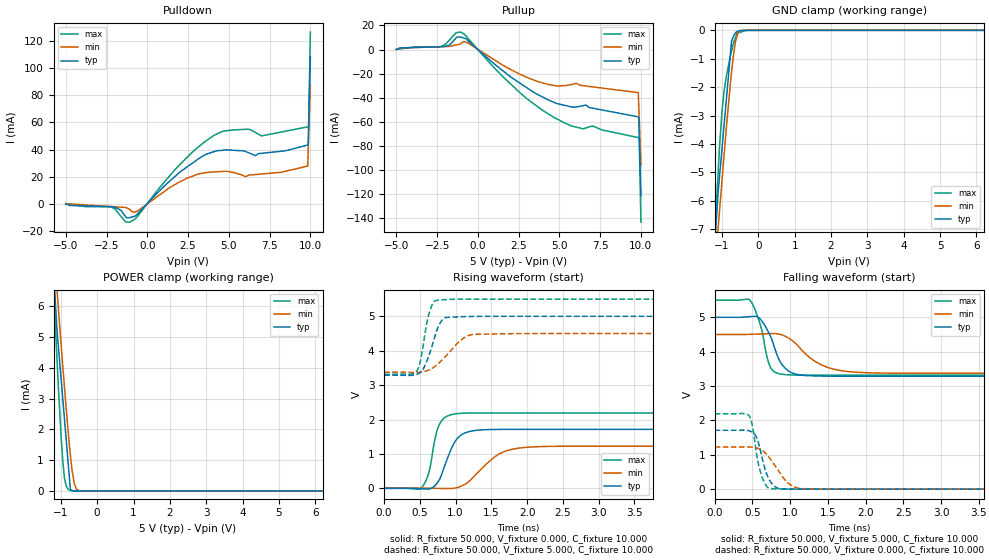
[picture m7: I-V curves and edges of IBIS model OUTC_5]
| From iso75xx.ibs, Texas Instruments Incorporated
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|   OUTC_5 MODEL
[Model]   OUTC_5
Model_type   3-state
Polarity   Non-Inverting
Vmeas = 2.5
Vref = 2.5
Cref = 15pF
Rref = 50
|   typ   min   max
| High state   (typ PVT)   (Fast PVT)  (Slow PVT)
C_comp   1.5194p   1.2464p   1.8503p
|C_comp (Low state)   1.4779p   1.2343p   1.7765p
[Voltage Range]   5   4.5   5.5
[Temperature Range]   27   125   -40
[Pullup Reference]   5   4.5   5.5
[Pulldown Reference]   -0   -0   -0
[Power Clamp Reference]   5   4.5   5.5
[GND Clamp Reference]   -0   -0   -0
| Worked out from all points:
|   slope of the pulldown table from 0 to 0.75 V, typ, clamps not added: 79.5 ohm
|   slope of the pullup table from 0 to 0.75 V, typ, clamps not added: 84.1 ohm
|   GND clamp passes 1 mA (typ) near -0.78 V on its own axis
|   POWER clamp passes 1 mA (typ) near -0.80 V on its own axis
|   falling waveform, R_fixture 50.000, V_fixture 5.000, C_fixture 10.000: 20-80 % time 200ps typ, 381ps min, 143ps max; typ from 5 V to 3.29 V
|   rising waveform, R_fixture 50.000, V_fixture 0.000, C_fixture 10.000: 20-80 % time 202ps typ, 383ps min, 130ps max; typ from 0 V to 1.71 V
|   rising waveform, R_fixture 50.000, V_fixture 5.000, C_fixture 10.000: 20-80 % time 166ps typ, 311ps min, 114ps max; typ from 3.29 V to 5 V
|   falling waveform, R_fixture 50.000, V_fixture 0.000, C_fixture 10.000: 20-80 % time 132ps typ, 241ps min, 108ps max; typ from 1.71 V to 0 V
[Pulldown]
|   Voltage   I(typ)   I(min)   I(max)
-5V       -93.83uA   -72.15uA   -88.32uA
-2.275V   -2.321mA   -2.154mA   -2.283mA
-1.07V    -10.42mA   -4.455mA   -13.77mA
-627mV    -8.011mA   -5.787mA   -9.836mA
2.106V    24.33mA    16.74mA    30.13mA
4.14V     38.62mA    23.45mA    50.79mA
6.625V    35.45mA    21.48mA    52.63mA
7.006V    37.17mA    21.87mA    50.06mA
9.838V    43.29mA    27.78mA    56.76mA
9.862V    43.37mA    36.98mA    56.82mA
9.896V    59.33mA    49.4mA     56.89mA
10V       108.8mA    87.9mA     126.9mA
[GND Clamp]
|   Voltage   I(typ)   I(min)   I(max)
-5V       -63.94mA   -55.54mA   -73.03mA
-1.935V   -22.09mA   -20.21mA   -25.09mA
-1.103V   -5.671mA   -6.938mA   -4.97mA
-1.07V    -5.19mA    -6.406mA   -4.162mA
-996.5mV  -4.13mA    -5.245mA   -2.82mA
-947.5mV  -3.424mA   -4.484mA   -2.199mA
-737.3mV  -392.9uA   -1.49mA    -732.2uA
-627mV    -92.24uA   -380.6uA   -251.3uA
-588.1mV  -39.49uA   -213.3uA   -113.7uA
-494.5mV  -4.813uA   -17.86uA   -65.8uA
-345.8mV  -3.447uA   -354.9nA   -2.997uA
10V       0A         0A         0A
[Pullup]
|   Voltage   I(typ)   I(min)   I(max)
-5V       96.38uA    77.66uA    98.88uA
-2.321V   2.306mA    2.381mA    2.34mA
-1.07V    10.35mA    4.74mA     14.49mA
-627mV    7.651mA    5.699mA    9.647mA
2.682V    -28.79mA   -21.05mA   -37.03mA
4.702V    -43.94mA   -29.85mA   -56.47mA
6.43V     -46.56mA   -29.87mA   -65.77mA
7.006V    -48.49mA   -30.86mA   -63.32mA
9.838V    -55.77mA   -35.71mA   -72.96mA
9.862V    -55.83mA   -44.87mA   -73.03mA
9.896V    -71.75mA   -57.24mA   -73.12mA
10V       -121mA     -95.55mA   -143.1mA
[POWER Clamp]
|   Voltage   I(typ)   I(min)   I(max)
-5V       63.78mA    55.35mA    72.89mA
-1.896V   20.91mA    19.19mA    23.74mA
-1.103V   5.222mA    6.529mA    4.274mA
-1.084V   4.953mA    6.225mA    3.806mA
-996.5mV  3.713mA    4.845mA    1.876mA
-947.5mV  3.022mA    4.091mA    999.2uA
-898.6mV  2.33mA     3.356mA    411.6uA
-751.6mV  256uA      1.338mA    17.39uA
-737.3mV  53.36uA    1.18mA     14.19uA
-627mV    2.548uA    222.8uA    1.235uA
-494.5mV  41.82nA    7.084uA    67.6nA
10V       0A         0A         0A
[Ramp]
R_load = 50
|   typ   min   max
dV/dt_r   1.04753/2.02389e-10   0.742676/3.83734e-10   1.35204/1.29551e-10
dV/dt_f   1.04642/1.9958e-10   0.677925/3.80599e-10   1.34435/1.43063e-10
[Falling Waveform]
R_fixture = 50.000
V_fixture = 5.000
V_fixture_min = 4.500
V_fixture_max = 5.500
C_fixture = 10.000
|  time   V(typ)   V(min)   V(max)
0s        5V         4.5V       5.5V
464.6ps   5.019V     4.504V     5.501V
598.6ps   4.956V     4.515V     4.823V
728.2ps   4.5V       4.524V     3.597V
783.5ps   4.182V     4.526V     3.422V
877.7ps   3.673V     4.496V     3.348V
1.08ns    3.342V     4.226V     3.319V
1.411ns   3.29V      3.619V     3.315V
1.783ns   3.285V     3.418V     3.315V
6ns       3.285V     3.37V      3.316V
[Rising Waveform]
R_fixture = 50.000
V_fixture = 0.000
V_fixture_min = 0.000
V_fixture_max = 0.000
C_fixture = 10.000
|  time   V(typ)   V(min)   V(max)
0s        -125.9uV   8.032mV    34.52uV
531.1ps   -13.86mV   5.666mV    34.22mV
624.5ps   -19mV      3.109mV    448.1mV
709.8ps   75.4mV     -3.951uV   1.417V
765ps     223.2mV    -2.021mV   1.821V
970.8ps   1.287V     2.247mV    2.155V
1.216ns   1.662V     258mV      2.189V
1.606ns   1.712V     995.4mV    2.191V
1.881ns   1.714V     1.168V     2.191V
6ns       1.713V     1.225V     2.191V
[Rising Waveform]
R_fixture = 50.000
V_fixture = 5.000
V_fixture_min = 4.500
V_fixture_max = 5.500
C_fixture = 10.000
|  time   V(typ)   V(min)   V(max)
0s        3.285V     3.374V     3.314V
451.4ps   3.307V     3.367V     3.392V
504.5ps   3.364V     3.375V     3.675V
624.5ps   3.846V     3.437V     5.05V
672.4ps   4.15V      3.488V     5.336V
728.2ps   4.535V     3.571V     5.462V
849.3ps   4.954V     3.812V     5.484V
1.083ns   4.987V     4.324V     5.498V
1.257ns   4.996V     4.473V     5.499V
6ns       5V         4.5V       5.5V
[Falling Waveform]
R_fixture = 50.000
V_fixture = 0.000
V_fixture_min = 0.000
V_fixture_max = 0.000
C_fixture = 10.000
|  time   V(typ)   V(min)   V(max)
0s        1.713V     1.226V     2.194V
451.4ps   1.7V       1.228V     2.148V
504.5ps   1.647V     1.219V     1.799V
557.6ps   1.49V      1.199V     977.3mV
598.6ps   1.191V     1.167V     562.3mV
661.1ps   631.6mV    1.077V     182.2mV
728.2ps   260.3mV    902.5mV    22.32mV
944.6ps   9.369mV    238.5mV    1.671mV
1.153ns   1.604mV    17.62mV    329.8uV
6ns       2.394nV    5.094nV    4.914nV
